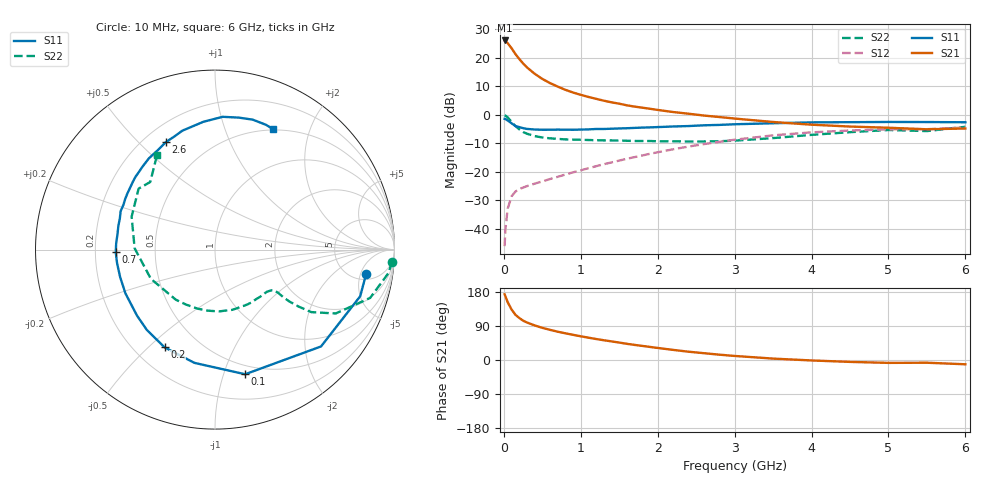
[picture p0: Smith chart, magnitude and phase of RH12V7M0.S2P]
! SIEMENS Small Signal Semiconductors
! BFR106
! Si NPN RF Bipolar Junction Transistor in SOT23
! VCE = 12 V  IC = 7 mA
! Common Emitter S-Parameters:  August  1996
# GHz  S  MA  R  50
!  f  S11  S21  S12  S22
! GHz  MAG  ANG  MAG  ANG  MAG  ANG  MAG  ANG
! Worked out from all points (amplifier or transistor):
!   36 points, 10 MHz to 6 GHz, reference 50 ohm
!   highest |S21| = 26.1 dB at 10 MHz (marker M1)
!   |S21| within 3 dB of that: start of sweep to 107 MHz
!   unconditionally stable (mu >= 1): 572.1 MHz to 1.922 GHz; 5.169 GHz to end of sweep
!   at 250 MHz: K = 0.59, MSG = 21.8 dB, |S12| = -25.4 dB
!   at 1.4 GHz: K = 1.12, MAG = 8.4 dB, |S12| = -16.6 dB
!   at 6 GHz: K = 1.01, MAG = -0.9 dB, |S12| = -4.4 dB
!   S11 on the Smith chart (normalised r, x): 10 MHz: 6.39, -6.27; 100 MHz: 0.42, -1.18; 200 MHz: 0.32, -0.56; 700 MHz: 0.29, -0.01; 2.6 GHz: 0.29, +0.60; 6 GHz: 0.49, +1.48
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0.01  0.8532 -9.0  20.25 173.4  0.005 88.0  0.9888 -3.9
0.02  0.8497 -17.8  20 168.4  0.0097 80.4  0.9762 -7.6
0.05  0.8001 -42.4  18.13 152.5  0.0227 68.8  0.9053 -17.3
0.1  0.7145 -76.4  14.82 133.4  0.0374 55.8  0.7608 -27.9
0.15  0.6414 -100.3  11.72 119.5  0.0453 47.6  0.6394 -33.0
0.2  0.6128 -117.3  9.608 110.9  0.0498 45.2  0.5614 -34.3
0.25  0.587 -130.3  8.008 103.9  0.0534 43.7  0.5035 -34.9
0.3  0.5694 -139.7  6.835 99.0  0.0564 44.3  0.4692 -34.9
0.4  0.5554 -154.0  5.288 91.3  0.0624 46.4  0.4258 -34.4
0.5  0.5503 -163.8  4.287 84.9  0.0683 48.9  0.4027 -34.5
0.6  0.5508 -172.1  3.623 79.6  0.0752 51.6  0.3894 -35.6
0.7  0.5532 -178.4  3.143 74.7  0.0822 54.6  0.3803 -37.3
0.9  0.5501 171.1  2.474 66.4  0.0986 58.5  0.3694 -40.8
1.1  0.5582 161.7  2.071 58.9  0.1165 61.4  0.3637 -46.3
1.3  0.5678 154.0  1.779 52.1  0.1368 63.1  0.358 -52.0
1.6  0.5852 144.0  1.475 42.7  0.1704 64.0  0.3526 -62.2
2.2  0.6277 126.0  1.126 26.7  0.2501 61.0  0.3452 -86.5
2.6  0.6585 114.6  0.977 18.0  0.3078 56.3  0.3432 -106.3
3.5  0.7151 95.2  0.753 3.7  0.4392 41.7  0.3927 -155.5
4.5  0.7473 79.7  0.626 -5.0  0.5341 22.6  0.4993 158.5
5.5  0.7511 67.8  0.561 -7.2  0.5634 9.5  0.5215 133.8
6  0.7448 64.1  0.579 -11.3  0.6038 1.4  0.6198 121.3
